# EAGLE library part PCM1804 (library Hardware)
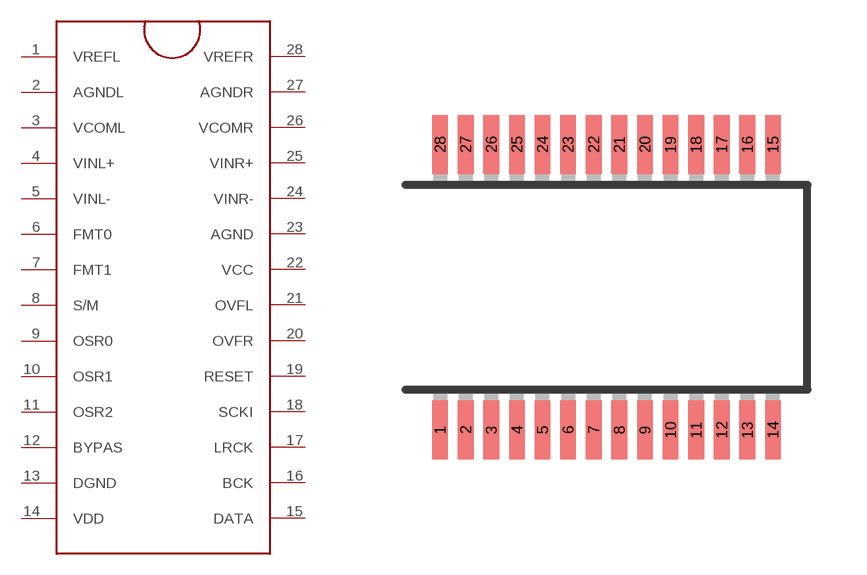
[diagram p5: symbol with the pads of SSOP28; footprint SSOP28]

Designator prefix -

## PCM1804  [SSOP28]
1  VREFL
2  AGNDL
3  VCOML
4  VINL+
5  VINL-
6  FMT0
7  FMT1
8  S/M
9  OSR0
10  OSR1
11  OSR2
12  BYPAS
13  DGND
14  VDD
15  DATA
16  BCK
17  LRCK
18  SCKI
19  RESET
20  OVFR
21  OVFL
22  VCC
23  AGND
24  VINR-
25  VINR+
26  VCOMR
27  AGNDR
28  VREFR

## Footprint SSOP28 (pad centres in mm)
Shrink Small Outline Package package type SS
smd 0.4 x 1.5: 1 -4.225,-3.625; 2 -3.575,-3.625; 3 -2.925,-3.625; 4 -2.275,-3.625; 5 -1.625,-3.625; 6 -0.975,-3.625; 7 -0.325,-3.625; 8 0.325,-3.625; 9 0.975,-3.625; 10 1.625,-3.625; 11 2.275,-3.625; 12 2.925,-3.625; 13 3.575,-3.625; 14 4.225,-3.625; 15 4.225,3.625; 16 3.575,3.625; 17 2.925,3.625; 18 2.275,3.625; 19 1.625,3.625; 20 0.975,3.625; 21 0.325,3.625; 22 -0.325,3.625; 23 -0.975,3.625; 24 -1.625,3.625; 25 -2.275,3.625; 26 -2.925,3.625; 27 -3.575,3.625; 28 -4.225,3.625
